FUNCTION_BLOCK Axis_PTP_CoE
VAR_INPUT
	Execute:				BOOL;
	bReset:					BOOL;
	Ref:					AXIS_REF;
	IO:						Axis_IO;
	mcJog:					MC_Jog;
	mcHome:					FB_Home_ByLimit;
	mcMoveAbsolute:			MC_MoveAbsolute;
	mcMoveRelative:			MC_MoveRelative;
	mcMoveVelocity:			MC_MoveVelocity;
	mcSoEReset:				FB_SoEReset;
	mcPower:				MC_Power;
	mcReset:				MC_Reset;
	mcStop:					MC_Stop;

	Target					:	LREAL;
	Velo					: 	LREAL;
	Jerk					:	LREAL := 0.0;
	Acc						:	LREAL := 0.0;
	Dec						:	LREAL := 0.0;

	sName:					WSTRING:="轴";
END_VAR
VAR
	Done:					BOOL;(*功能块执行完成状态*)
	Busy: 					BOOL;(*功能块正在执行状态*)
	Active:					BOOL;
	CommandAborted:			BOOL;
	Error:					BOOL;
	ErrorID:				UDINT;
END_VAR

;

ACTION aHome:
(*
TYPE MC_HomingMode :
(
	MC_DefaultHoming,		(* default homing as defined in the SystemManager encoder parameters *)
	MC_AbsSwitch, 		(* not implemented - Absolute Switch homing plus Limit switches *)
	MC_LimitSwitch, 		(* not implemented - Homing against Limit switches *)
	MC_RefPulse, 		(* not implemented - Homing using encoder Reference Pulse "Zero Mark" *)
	MC_Direct, 		(* Static Homing forcing position from user reference *)
	MC_Absolute, 		(* not implemented - Static Homing forcing position from absolute encoder *)
	MC_Block, 		(* not implemented - Homing against hardware parts blocking movement *)
	MC_ForceCalibration, 	(* set the calibration flag without performing any motion or changing the position *)
	MC_ResetCalibration  	(* resets the calibration flag without performing any motion or changing the position *)
);
END_TYPE

*)


mcHome(
	Execute:= 			Execute,
	Position:= 			,
	HomingMode:= 		,
	PosLimit:=			IO.snLimitP,
	NegLimit:=			IO.snLimitN,
	bCalibrationCam:= 	IO.snHome,
	Axis:= 				Ref,
	Done=>				Done,
	Busy=> 			Busy,
	Active=> 		Active,
	CommandAborted=> CommandAborted,
	Error=> 		Error,
	ErrorID=> 		ErrorID
	);
END_ACTION

ACTION aIO:
IO.DriverDI();(*调用axis_io*)

IO.snLimitP	:=IO.DriverDI.bLimitSenser_P;
IO.snLimitN	:=IO.DriverDI.bLimitSenser_N;
IO.snHome	:=IO.DriverDI.bHomeSenser;


IF IO.snLimitP
OR IO.snLimitN THEN(*极限*)
	DATA.Motor_Limit:=TRUE;
END_IF

IF IO.DriverDI.bHwError THEN(*×硬件故障*)
	DATA.Motor_HwError:=TRUE;
END_IF

IF Ref.Status.Error THEN(*NC的故障状态*)
	DATA.Motor_SwError:=TRUE;
	DATA.Motor_SwErrId:=Ref.Status.ErrorID;
	
END_IF
END_ACTION

ACTION aJogB:
mcJog(
	JogForward:= 	FALSE,
	JogBackwards:= 	Execute,
	Mode:= 			MC_JOGMODE_CONTINOUS,
	Position:= 		,
	Velocity:= 		Velo,
	Acceleration:= 	Acc,
	Deceleration:= 	Dec,
	Jerk:= 			Jerk,
	Axis:= 			Ref,
	Busy=> 			Busy,
	Active=> 		Active,
	CommandAborted=> CommandAborted,
	Error=> 		Error,
	ErrorID=> 		ErrorID
	);
END_ACTION

ACTION aJogF:
mcJog(
	JogForward:= 	Execute,
	JogBackwards:= 	FALSE,
	Mode:= 			MC_JOGMODE_CONTINOUS,
	Position:= 		,
	Velocity:= 		Velo,
	Acceleration:= 	Acc,
	Deceleration:= 	Dec,
	Jerk:= 			Jerk,
	Axis:= 			Ref,
	Busy=> 			Busy,
	Active=> 		Active,
	CommandAborted=> CommandAborted,
	Error=> 		Error,
	ErrorID=> 		ErrorID
	);
END_ACTION

ACTION aManualJOG:
(*
TYPE E_JogMode :
(
	MC_JOGMODE_STANDARD_SLOW, (* motion with standard jog parameters for slow motion *)
	MC_JOGMODE_STANDARD_FAST, (* motion with standard jog parameters for fast motion *)
	MC_JOGMODE_CONTINOUS,     (* axis moves as long as the jog button is pressed using parameterized dynamics *)
	MC_JOGMODE_INCHING,       (* axis moves for a certain relative distance *)
	MC_JOGMODE_INCHING_MODULO (* axis moves for a certain relative distance - stop position is rounded to the distance value *)
);
END_TYPE

*)

mcJog(
	JogForward:= 	IO.btManualJogF,
	JogBackwards:= 	IO.btManualJogB,
	Mode:= 			MC_JOGMODE_CONTINOUS,
	Position:= 		,
	Velocity:= 		Velo,
	Acceleration:= 	Acc,
	Deceleration:= 	Dec,
	Jerk:= 			Jerk,
	Axis:= 			Ref,
	Busy=> 			Busy,
	Active=> 		Active,
	CommandAborted=> CommandAborted,
	Error=> 		Error,
	ErrorID=> 		ErrorID
	);
END_ACTION

ACTION aMoveAbs:
mcMoveAbsolute(
	Execute:= 		Execute,
	Position:= 		Target,
	Velocity:= 		Velo,
	Acceleration:= 	Acc,
	Deceleration:= 	Dec,
	Jerk:= 			Jerk,
	Axis:= 			Ref,
	Done=> 			Done,
	Busy=> 			Busy,
	Active=> 		Active,
	CommandAborted=> CommandAborted,
	Error=> 		Error,
	ErrorID=> 		ErrorID
	);
END_ACTION

ACTION aMoveOff:
(*触发条件复位*)
mcHome(
	Execute:= 		FALSE,
	Axis:= 			Ref,
	);

mcJog(
	JogForward:= 	FALSE,
	JogBackwards:= 	FALSE,
	Axis:= 			Ref,
	);

mcMoveAbsolute(
	Execute:= 		FALSE,
	Axis:= 			Ref,
	);

mcMoveRelative(
	Execute:= 		FALSE,
	Axis:= 			Ref,
	);

mcMoveVelocity(
	Execute:= 		FALSE,
	Axis:= 			Ref,
	);

Done:=FALSE;
Busy:=FALSE;
Active:=FALSE;
CommandAborted:=FALSE;
Error:=FALSE;
END_ACTION

ACTION aMoveRel:
mcMoveRelative(
	Execute:= 		Execute,
	Distance:= 		Target,
	Velocity:= 		Velo,
	Acceleration:= 	Acc,
	Deceleration:= 	Dec,
	Jerk:= 			Jerk,
	Axis:= 			Ref,
	Done=> 			Done,
	Busy=> 			Busy,
	Active=> 		Active,
	CommandAborted=> CommandAborted,
	Error=> 		Error,
	ErrorID=> 		ErrorID
	);
END_ACTION

ACTION aMoveVel:
mcMoveVelocity(
	Execute:= 		Execute,
	Direction:= 	,
	Velocity:= 		Velo,
	Acceleration:= 	Acc,
	Deceleration:= 	Dec,
	Jerk:= 			Jerk,
	Axis:= 			Ref,
	InVelocity=> 	Done,
	Busy=> 			Busy,
	Active=> 		Active,
	CommandAborted=> CommandAborted,
	Error=> 		Error,
	ErrorID=> 		ErrorID );
END_ACTION

ACTION aPower:
mcPower(
	Enable:= 			TRUE,
	Enable_Positive:= true	,
	Enable_Negative:=true 	,
	Override:= 		,
	BufferMode:= 	,
	Axis:= 			Ref,
	Status=> 		,
	Busy=> 			Busy,
	Active=> 		Active,
	Error=> 		Error,
	ErrorID=> 		ErrorID
	);
END_ACTION

ACTION aReset:
aIO();(*硬件IO刷新*)
Ref.ReadStatus();(*轴状态字刷新*)



(*NC复位*)
mcReset(
	Execute:= 	(bReset OR DATA.ResetAlarm)
				AND Ref.Status.Error,
	Axis:= 		Ref,
	);
(*AX5000驱动器复位*)
mcSoeReset(
	Execute:= 	(bReset OR DATA.ResetAlarm)
				AND Ref.Status.Error,
	Axis:= 		Ref,
	);


(*遇极限后禁止往极限方向运行*)
mcPower(
	Enable:= 			,
	Enable_Positive:= 	NOT IO.snLimitP
						
						AND mcPower.Enable,
	Enable_Negative:= 	NOT IO.snLimitN
					
						AND mcPower.Enable,
	Override:= 		,
	Axis:= 			Ref,

	);
END_ACTION

ACTION aStop:
aMoveOff(); (*触发条件复位*)
 
mcStop(
	Execute:= 		Execute,
	Deceleration:= 	Dec,
	Jerk:= 			Jerk,
	Options:= 		,
	Axis:= 			Ref,
	Done=> 			Done,
	Busy=> 			Busy,
	Active=> 		Active,
	CommandAborted=> CommandAborted,
	Error=> 		Error,
	ErrorID=> 		ErrorID
	);
END_ACTION

END_FUNCTION_BLOCK
